| TEXAS INSTRUMENTS INCORPORATED
| Standard Linear and Logic Group
| IBIS Model of SN74CB3T3245
| 3.3V LOW-VOLTAGE OCTAL FET BUS SWITCH WITH 5V TOLERANT/LEVEL SHIFTER
| This file contains package information for the following:
|  SSOP 20-pin (DBQ) package as [Component] CB3T3245_DBQ
|  TVSOP 20-pin (DGV) package as [Component] CB3T3245_DGV
|  SOIC 20-pin (DW) package as [Component] CB3T3245_DW
|  TSSOP 20-pin (PW) package as [Component] CB3T3245_PW
| This device can be powered at the following Vccs:
|  3.3 volt Vcc
|  2.5 volt Vcc
| This file provides unique models under the [Model Selector] for each Vcc.
| For operation at a specific Vcc, select the appropriate model after each
| [Model Selector] keyword.
[IBIS Ver]   3.2
[Comment char]  |_char
[File Name]   sn74cb3t3245.ibs
[File Rev]   1.1 | x_die
[Date]   July 30, 2003
[Source]   Data created from TI-SPICE simulations at TI-SLL.
[Notes]   The following is an IBIS list for the CB3T3245.
   Please contact sllibis@ti.com with questions and
   comments concerning SLL IBIS models.
   - Power-clamp data has been deleted since there is no
   power-clamp diode in the device.
   - Non-monotonic data due to FET characteristics.
[Disclaimer] Property of Texas Instruments Incorporated.  Unauthorized
   reproduction and/or distribution is strictly prohibited.
   This product is protected under copyright law.
   Created  2003, (C) Copyright  2003, Texas Instruments
   Incorporated, All Rights Reserved
   UNLESS THERE IS A SIGNED, WRITTEN AGREEMENT TO THE
   CONTRARY, TEXAS INSTRUMENTS (TI) IS PROVIDING THE IBIS
   MODELS  AND WITHOUT ANY WARRANTY, EXPRESSED OR
   IMPLIED.  TI assumes no liability for:
   1) the accuracy of the IBIS models provided to your
   company;
   2) the proper functioning of these IBIS Models in your
   design or for any resulting applications; or
   3) infringement of patents, copyrights or intellectual
   property rights resulting from your use of these IBIS
   models.
   TI provides IBIS Models as a service to our customers.
   You and your company shall not distribute, sell or give
   these models to anyone else without prior written
   permission from TI.
   TI reserves the right to make changes to our products or
   to discontinue any semiconductor product or service
   without notice, and advises our customers to obtain the
   latest version of relevant information to verify, before
   placing orders, that the information being relied on is
   current.
   Please be aware that your receipt and use of the IBIS
   information provided shall serve as acceptance of these
   terms and conditions.  If you do not accept these terms,
   you should return or destroy the IBIS models and any
   other accompanying information immediately.
| Component CB3T3245_DBQ 20-pin SSOP
[Component]   CB3T3245_DBQ
[Manufacturer]   Texas Instruments, Inc.
[Package]
|   typ   min   max
R_pkg   3.900e-02   3.100e-02   5.000e-02
L_pkg   2.804e-09   2.292e-09   3.805e-09
C_pkg   2.940e-13   2.220e-13   4.170e-13
[Pin]   signal_name   model_name   R_pin   L_pin   C_pin
1   NC   NC   4.800e-02   3.760e-09   4.140e-13
2   A1   CB3T3245_IO   4.800e-02   3.053e-09   3.500e-13
3   A2   CB3T3245_IO   3.500e-02   2.506e-09   2.530e-13
4   A3   CB3T3245_IO   3.300e-02   2.368e-09   2.250e-13
5   A4   CB3T3245_IO   3.200e-02   2.302e-09   2.260e-13
6   A5   CB3T3245_IO   3.200e-02   2.303e-09   2.260e-13
7   A6   CB3T3245_IO   3.300e-02   2.368e-09   2.250e-13
8   A7   CB3T3245_IO   3.500e-02   2.506e-09   2.530e-13
9   A8   CB3T3245_IO   4.800e-02   3.053e-09   3.490e-13
10   GND   GND   4.200e-02   3.572e-09   4.040e-13
11   B8   CB3T3245_IO   4.700e-02   3.731e-09   4.140e-13
12   B7   CB3T3245_IO   4.900e-02   3.095e-09   3.550e-13
13   B6   CB3T3245_IO   4.000e-02   2.616e-09   2.590e-13
14   B5   CB3T3245_IO   3.300e-02   2.336e-09   2.220e-13
15   B4   CB3T3245_IO   3.300e-02   2.292e-09   2.250e-13
16   B3   CB3T3245_IO   3.300e-02   2.313e-09   2.270e-13
17   B2   CB3T3245_IO   3.100e-02   2.350e-09   2.230e-13
18   B1   CB3T3245_IO   4.000e-02   2.630e-09   2.600e-13
19   NOE   CB3T3245_IN   4.900e-02   3.109e-09   3.550e-13
20   VCC   POWER   5.000e-02   3.805e-09   4.170e-13
| Component CB3T3245_DGV 20-pin TVSOP
[Component]   CB3T3245_DGV
[Manufacturer]   Texas Instruments, Inc.
[Package]
|   typ   min   max
R_pkg   4.400e-02   3.800e-02   4.800e-02
L_pkg   2.561e-09   2.236e-09   2.961e-09
C_pkg   3.420e-13   2.640e-13   4.460e-13
[Pin]   signal_name   model_name   R_pin   L_pin   C_pin
1   NC   NC   4.400e-02   2.935e-09   4.170e-13
2   A1   CB3T3245_IO   4.200e-02   2.869e-09   4.460e-13
3   A2   CB3T3245_IO   4.300e-02   2.399e-09   3.160e-13
4   A3   CB3T3245_IO   4.400e-02   2.236e-09   2.650e-13
5   A4   CB3T3245_IO   4.600e-02   2.278e-09   2.640e-13
6   A5   CB3T3245_IO   4.500e-02   2.274e-09   2.640e-13
7   A6   CB3T3245_IO   4.400e-02   2.285e-09   2.690e-13
8   A7   CB3T3245_IO   4.300e-02   2.452e-09   3.200e-13
9   A8   CB3T3245_IO   4.400e-02   2.900e-09   4.460e-13
10   GND   GND   4.400e-02   2.961e-09   4.180e-13
11   B8   CB3T3245_IO   4.500e-02   2.954e-09   4.180e-13
12   B7   CB3T3245_IO   4.200e-02   2.847e-09   4.430e-13
13   B6   CB3T3245_IO   4.500e-02   2.453e-09   3.190e-13
14   B5   CB3T3245_IO   4.500e-02   2.297e-09   2.690e-13
15   B4   CB3T3245_IO   4.800e-02   2.334e-09   2.680e-13
16   B3   CB3T3245_IO   4.800e-02   2.335e-09   2.670e-13
17   B2   CB3T3245_IO   4.600e-02   2.299e-09   2.680e-13
18   B1   CB3T3245_IO   4.600e-02   2.457e-09   3.200e-13
19   NOE   CB3T3245_IN   4.300e-02   2.848e-09   4.410e-13
20   VCC   POWER   3.800e-02   2.812e-09   4.080e-13
| Component CB3T3245_DW 20-pin SOIC
[Component]   CB3T3245_DW
[Manufacturer]   Texas Instruments, Inc.
[Package]
|   typ   min   max
R_pkg   3.800e-02   3.300e-02   4.500e-02
L_pkg   5.012e-09   4.110e-09   6.349e-09
C_pkg   7.170e-13   5.300e-13   8.680e-13
[Pin]   signal_name   model_name   R_pin   L_pin   C_pin
1   NC   NC   4.200e-02   6.336e-09   8.650e-13
2   A1   CB3T3245_IO   4.300e-02   5.542e-09   8.670e-13
3   A2   CB3T3245_IO   3.400e-02   4.714e-09   7.320e-13
4   A3   CB3T3245_IO   3.400e-02   4.377e-09   5.910e-13
5   A4   CB3T3245_IO   3.600e-02   4.130e-09   5.330e-13
6   A5   CB3T3245_IO   3.500e-02   4.111e-09   5.300e-13
7   A6   CB3T3245_IO   3.400e-02   4.284e-09   5.830e-13
8   A7   CB3T3245_IO   3.400e-02   4.634e-09   7.260e-13
9   A8   CB3T3245_IO   4.000e-02   5.518e-09   8.650e-13
10   GND   GND   4.300e-02   6.349e-09   8.660e-13
11   B8   CB3T3245_IO   4.100e-02   6.281e-09   8.610e-13
12   B7   CB3T3245_IO   4.500e-02   5.561e-09   8.680e-13
13   B6   CB3T3245_IO   3.300e-02   4.778e-09   7.420e-13
14   B5   CB3T3245_IO   3.500e-02   4.414e-09   5.960e-13
15   B4   CB3T3245_IO   3.500e-02   4.110e-09   5.330e-13
16   B3   CB3T3245_IO   3.600e-02   4.130e-09   5.330e-13
17   B2   CB3T3245_IO   3.400e-02   4.377e-09   5.910e-13
18   B1   CB3T3245_IO   3.400e-02   4.714e-09   7.310e-13
19   NOE   CB3T3245_IN   4.300e-02   5.569e-09   8.680e-13
20   VCC   POWER   4.200e-02   6.308e-09   8.640e-13
| Component CB3T3245_PW 20-pin TSSOP
[Component]   CB3T3245_PW
[Manufacturer]   Texas Instruments, Inc.
[Package]
|   typ   min   max
R_pkg   5.000e-02   4.200e-02   6.000e-02
L_pkg   2.802e-09   2.248e-09   3.553e-09
C_pkg   3.170e-13   2.020e-13   4.430e-13
[Pin]   signal_name   model_name   R_pin   L_pin   C_pin
1   NC   NC   5.500e-02   3.461e-09   4.400e-13
2   A1   CB3T3245_IO   5.500e-02   3.150e-09   4.010e-13
3   A2   CB3T3245_IO   4.200e-02   2.619e-09   3.020e-13
4   A3   CB3T3245_IO   4.500e-02   2.273e-09   2.020e-13
5   A4   CB3T3245_IO   4.500e-02   2.248e-09   2.240e-13
6   A5   CB3T3245_IO   4.500e-02   2.273e-09   2.260e-13
7   A6   CB3T3245_IO   4.400e-02   2.323e-09   2.050e-13
8   A7   CB3T3245_IO   4.600e-02   2.704e-09   3.070e-13
9   A8   CB3T3245_IO   6.000e-02   3.265e-09   4.110e-13
10   GND   GND   5.700e-02   3.506e-09   4.360e-13
11   B8   CB3T3245_IO   5.800e-02   3.553e-09   4.370e-13
12   B7   CB3T3245_IO   5.800e-02   3.193e-09   4.050e-13
13   B6   CB3T3245_IO   4.200e-02   2.704e-09   3.110e-13
14   B5   CB3T3245_IO   4.600e-02   2.392e-09   2.100e-13
15   B4   CB3T3245_IO   4.700e-02   2.334e-09   2.290e-13
16   B3   CB3T3245_IO   4.700e-02   2.300e-09   2.270e-13
17   B2   CB3T3245_IO   4.700e-02   2.349e-09   2.070e-13
18   B1   CB3T3245_IO   4.500e-02   2.677e-09   3.060e-13
19   NOE   CB3T3245_IN   6.000e-02   3.235e-09   4.060e-13
20   VCC   POWER   5.600e-02   3.487e-09   4.430e-13
[Series Switch Groups]
| Function Group States
On  1 /   | A1-A8->B1-B8 NOE LOW
Off  1 /   | A1-A8->B1-B8 NOE HIGH
[Series Pin Mapping]   pin_2   model_name   function_table_group
2   18   CB3T3245_IO_33_S   1
| 2   18   CB3T3245_IO_25_S   1
3   17   CB3T3245_IO_33_S   1
| 3   17   CB3T3245_IO_25_S   1
4   16   CB3T3245_IO_33_S   1
| 4   16   CB3T3245_IO_25_S   1
5   15   CB3T3245_IO_33_S   1
| 5   15   CB3T3245_IO_25_S   1
6   14   CB3T3245_IO_33_S   1
| 6   14   CB3T3245_IO_25_S   1
7   13   CB3T3245_IO_33_S   1
| 7   13   CB3T3245_IO_25_S   1
8   12   CB3T3245_IO_33_S   1
| 8   12   CB3T3245_IO_25_S   1
9   11   CB3T3245_IO_33_S   1
| 9   11   CB3T3245_IO_25_S   1
| Model CB3T3245_IN
[Model Selector]   CB3T3245_IN
CB3T3245_IN_33   3.3 volt Vcc
CB3T3245_IN_25   2.5 volt Vcc
| Model CB3T3245_IO
[Model Selector]   CB3T3245_IO
CB3T3245_IO_33   3.3 volt Vcc
CB3T3245_IO_25   2.5 volt Vcc
| Model CB3T3245_IO_S
[Model Selector]   CB3T3245_IO_S
CB3T3245_IO_33_S   3.3 volt Vcc
CB3T3245_IO_25_S   2.5 volt Vcc
[Model]   CB3T3245_IO_33_S
Model_type  Series_switch
| variable   typ   min   max
C_comp   0   0   0
[Temperature Range]   40   100   -40
| Ambient temperature   25   85   -40
[Voltage range]   3.3   3   3.6
[On]
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[Off]
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[Model]   CB3T3245_IO_25_S
Model_type  Series_switch
| variable   typ   min   max
C_comp   0   0   0
[Temperature Range]   40   100   -40
| Ambient temperature   25   85   -40
[Voltage range]   2.5   2.3   2.7
[On]
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[Off]
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| Models and submodels in the file (6): CB3T3245_IN_33 (Input), CB3T3245_IN_25 (Input), CB3T3245_IO_33_S (Series_switch), CB3T3245_IO_33 (Terminator), CB3T3245_IO_25_S (Series_switch), CB3T3245_IO_25 (Terminator)
